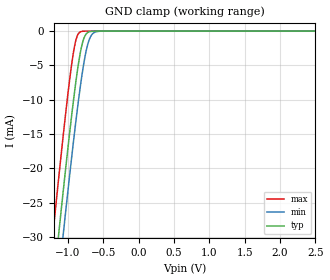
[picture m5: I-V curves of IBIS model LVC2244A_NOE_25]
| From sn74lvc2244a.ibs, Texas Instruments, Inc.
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[Model]   LVC2244A_NOE_25
Model_type  Input
Vinl=0.7
Vinh=1.7
| variable   typ   min   max
C_comp   5.31pF   4.85pF   5.83pF
[Temperature Range]   40   100   -40
| Ambient temperature   25   85   -40
[Voltage range]   2.5   2.3   2.7
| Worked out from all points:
|   GND clamp passes 1 mA (typ) near -0.77 V on its own axis
[GND Clamp]
| LVC2244A_NOE_25
|   Voltage   I(typ)   I(min)   I(max)
-5V       -443mA     -448.4mA   -436.3mA
-1.23V    -39.45mA   -45.8mA    -31.31mA
-1.205V   -36.93mA   -43.28mA   -28.78mA
-1.13V    -29.46mA   -35.8mA    -21.3mA
-1.07V    -23.6mA    -29.93mA   -15.5mA
-1.05V    -21.69mA   -27.99mA   -13.61mA
-955mV    -12.94mA   -19.06mA   -5.398mA
-885mV    -7.147mA   -12.88mA   -1.216mA
-780mV    -1.214mA   -4.964mA   -14.58uA
-715mV    -173.8uA   -1.747mA   -688.1nA
-645mV    -15.72uA   -327uA     -25.52nA
2.5V      7.132pA    13.06pA    6.802pA
